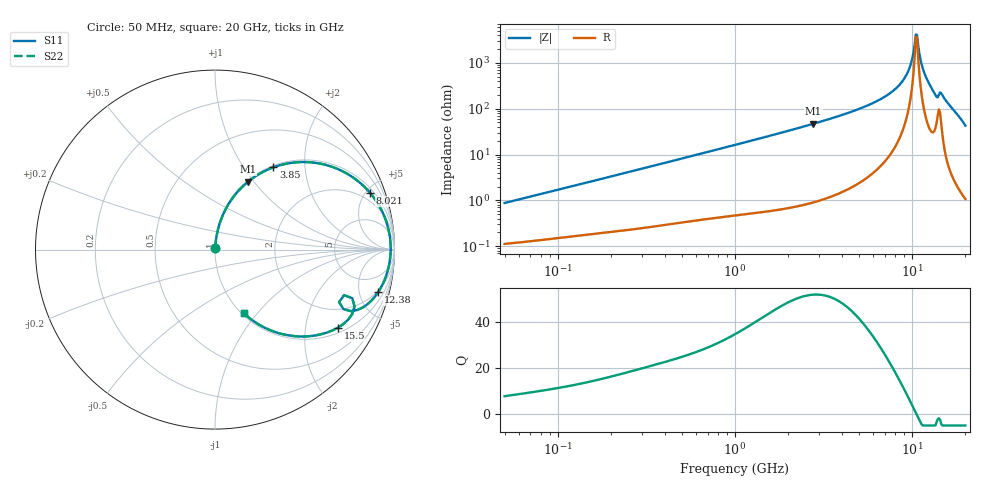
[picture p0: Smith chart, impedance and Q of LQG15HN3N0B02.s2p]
!Murata Part Number: LQG15HN3N0B02
!These Parameters are Measured in Series Mode Connection
!  o--[Z]--o
!Port1  Port2
!  o-------o
!Freq. Start=50[MHz] Stop=20[GHz], 401[Steps]
# Hz S RI R 50
!Freq.(Hz) S11(Real) S11(Imag) S21(Real) S21(Imag) S12(Real) S12(Imag) S22(Real) S22(Imag)
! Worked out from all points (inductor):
!   401 points, 50 MHz to 20 GHz, reference 50 ohm
!   read as one part in series: L = 2.74 nH near 51.52 MHz
!   highest Q = 51.9 at 2.769 GHz (marker M1), where L = 2.69 nH
!   self-resonance near 10.5 GHz
!   S11 on the Smith chart (normalised r, x): 50 MHz: 1.00, +0.02; 3.85 GHz: 1.03, +1.38; 8.021 GHz: 1.29, +5.32; 12.38 GHz: 1.82, -7.38; 15.5 GHz: 1.18, -3.01; 20 GHz: 1.02, -0.85
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5e7  0.00119 0.00866  0.9988 -0.00866  0.9988 -0.00866  0.00119 0.00866
1.364002e8  0.00224 0.0228  0.9978 -0.0228  0.9978 -0.0228  0.00224 0.0228
3.721004e8  0.00644 0.0604  0.9936 -0.0604  0.9936 -0.0604  0.00644 0.0604
1e9  0.0298 0.1562  0.9702 -0.1562  0.9702 -0.1562  0.0298 0.1562
2.728004e9  0.1793 0.3741  0.8207 -0.3741  0.8207 -0.3741  0.1793 0.3741
2.769174e9  0.1842 0.3781  0.8158 -0.3781  0.8158 -0.3781  0.1842 0.3781
3.850025e9  0.3253 0.4584  0.6747 -0.4584  0.6747 -0.4584  0.3253 0.4584
5.598765e9  0.5767 0.4808  0.4233 -0.4808  0.4233 -0.4808  0.5767 0.4808
7.442007e9  0.8076 0.3727  0.1924 -0.3727  0.1924 -0.3727  0.8076 0.3727
8.020766e9  0.8635 0.3169  0.1365 -0.3169  0.1365 -0.3169  0.8635 0.3169
9.457416e9  0.9567 0.1483  0.0433 -0.1483  0.0433 -0.1483  0.9567 0.1483
9.892087e9  0.9708 0.0918  0.0292 -0.0918  0.0292 -0.0918  0.9708 0.0918
1.034674e10  0.9781 0.0312  0.0219 -0.0312  0.0219 -0.0312  0.9781 0.0312
1.050288e10  0.9788 0.0102  0.0212 -0.0102  0.0212 -0.0102  0.9788 0.0102
1.082228e10  0.9773 -0.0328  0.0227 0.0328  0.0227 0.0328  0.9773 -0.0328
1.149051e10  0.9612 -0.1222  0.0388 0.1222  0.0388 0.1222  0.9612 -0.1222
1.238412e10  0.9095 -0.2364  0.0905 0.2364  0.0905 0.2364  0.9095 -0.2364
1.334722e10  0.7951 -0.3359  0.2049 0.3359  0.2049 0.3359  0.7951 -0.3359
1.438523e10  0.7647 -0.2706  0.2353 0.2706  0.2353 0.2706  0.7647 -0.2706
1.550395e10  0.6839 -0.4354  0.3161 0.4354  0.3161 0.4354  0.6839 -0.4354
1.747767e10  0.426 -0.4803  0.574 0.4803  0.574 0.4803  0.426 -0.4803
2e10  0.1601 -0.3543  0.8399 0.3543  0.8399 0.3543  0.1601 -0.3543
